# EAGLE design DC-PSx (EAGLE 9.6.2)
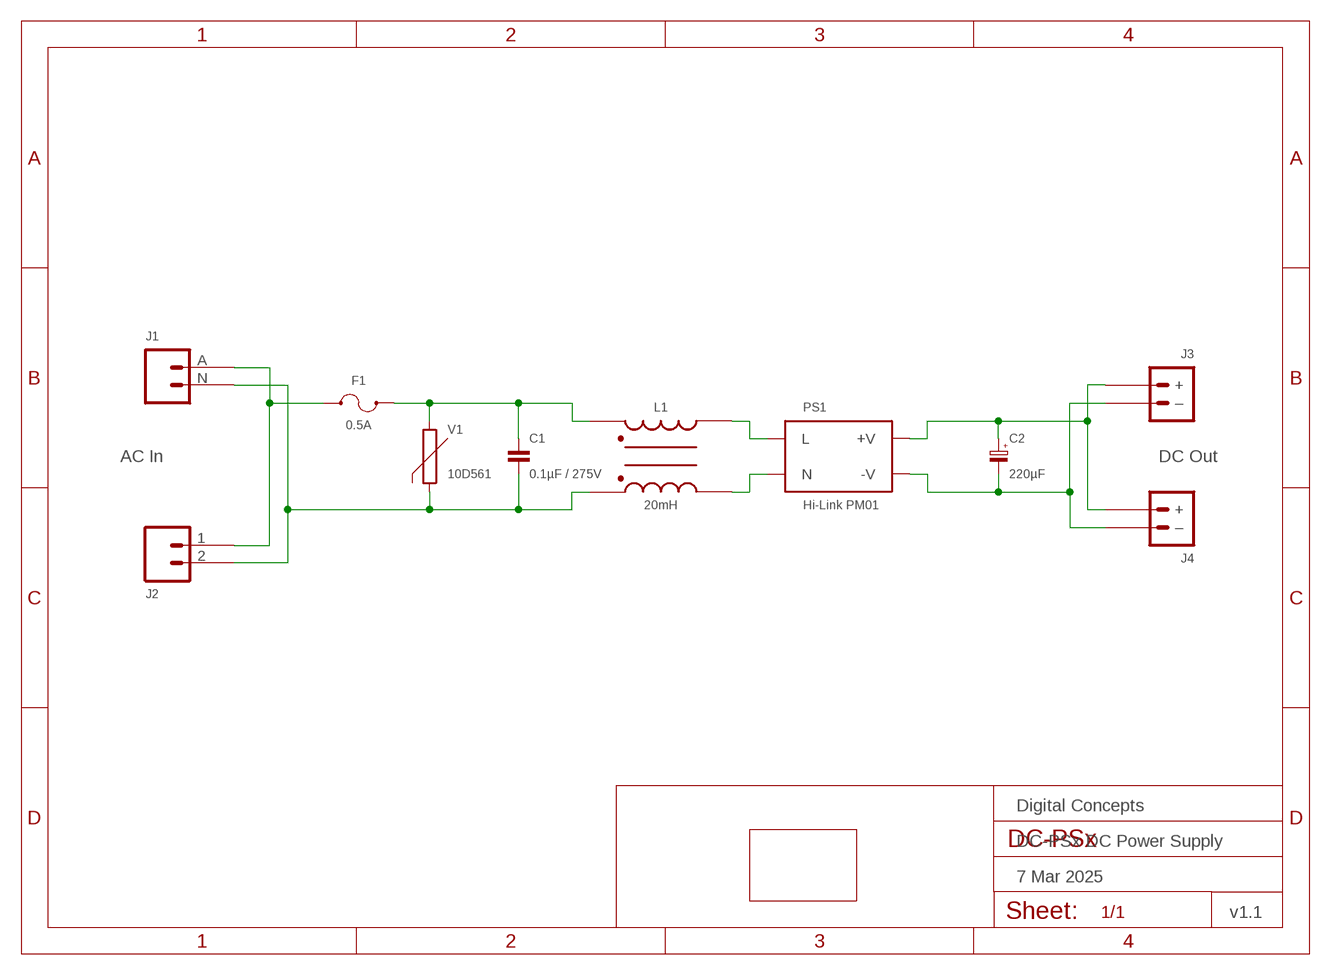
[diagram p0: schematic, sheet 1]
FRAME2 (FRAME_A5L-LOC): DATE: 7 Mar 2025; OWNER: Digital Concepts; TITLE: DC-PSx DC Power Supply; VERSION: v1.1

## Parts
C1  0.1µF / 275V  CAPACITOR-TENTA-SUPPRESSION  [CAPACITOR-TENTA-SUPPRESSION]
C2  220µF  CAPACITOR-ELECTROLYTICE5-10.5  [E5-10,5]
F1  0.5A  FUSE-HOLDER-1808  [FUSE-HOLDER-1808]
J1  AC In  AC_POWER_SOCKET_DB-03  [DB-03_AC_POWER_SOCKET]
J2  TERMINAL_SCREW_2P_VERTICAL  [TERMINAL-SCREW-2P]
J3  DC Out  JST-PH2.0-2-VERTICAL-POWER  [JST-PH2.0-2-VERTICAL-POWER]
J4  TERMINAL_SCREW_2P_POWER  [TERMINAL-SCREW-2P]
L1  20mH  INDUCTOR-COMMON-MODE-UU9.8  [INDUCTOR-UU9.8]
PCB1  PCB-OUTLINE-64X36  [PCB-POWER-SUPPLY-3]
PS1  Hi-Link PM01  POWER_SUPPLY-HI-LINK  [HI-LINK_PM0X]
V1  10D561  VARISTOR-10D561  [VARISTOR-10D561]

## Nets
N$1: F1.P$1 J1.A J2.1
N$2: C1.P$1 F1.P$2 L1.P$1 V1.2
N$3: L1.P$2 PS1.AC-L(L)
N$4: C1.P$2 J1.N J2.2 L1.P$4 V1.1
N$5: L1.P$3 PS1.AC-N(N)
N$6: C2.+ J3.+ J4.2(+) PS1.+VO(+V)
N$7: C2.- J3.-(–) J4.1(–) PS1.-VO(-V)

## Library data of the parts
C1 = digitalconcepts:CAPACITOR-TENTA-SUPPRESSION: MEX/TENTA Interference Suppression Capacitor
C2 = digitalconcepts:CAPACITOR-ELECTROLYTIC: Electrolytic Capacitor; SPICEPREFIX: C
F1 = digitalconcepts:FUSE-HOLDER-1808: 1808 Fuse Holder
J1 = digitalconcepts:AC_POWER_SOCKET_DB-03: DB-03 AC Power Socket
J2 = digitalconcepts:TERMINAL_SCREW_2P_VERTICAL: PCB Mount Screw-Type Terminal 2P
J3 = digitalconcepts:JST-PH2.0-2-VERTICAL-POWER: JST PH2.0 2P PTH Connector (Power)
J4 = digitalconcepts:TERMINAL_SCREW_2P_POWER: PCB Mount Screw-Type Terminal 2P
L1 = digitalconcepts:INDUCTOR-COMMON-MODE-UU9.8: UU9.8 Common Mode Inductor
PCB1 = digitalconcepts:PCB-OUTLINE-64X36: Power Supply PCB Outline (64 x 36)
PS1 = digitalconcepts:POWER_SUPPLY-HI-LINK: Hi-Link Power Supply Module
V1 = digitalconcepts:VARISTOR-10D561: VARISTOR

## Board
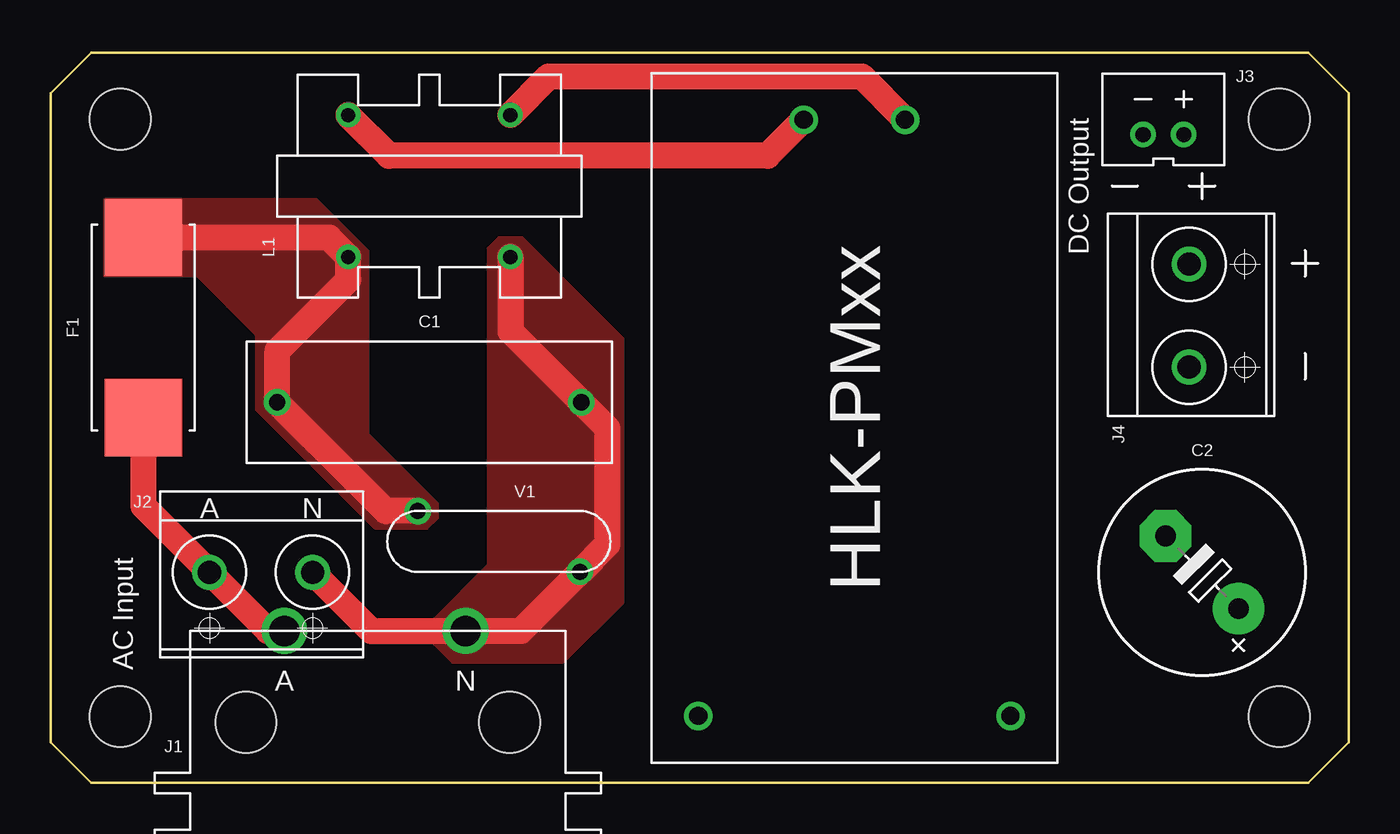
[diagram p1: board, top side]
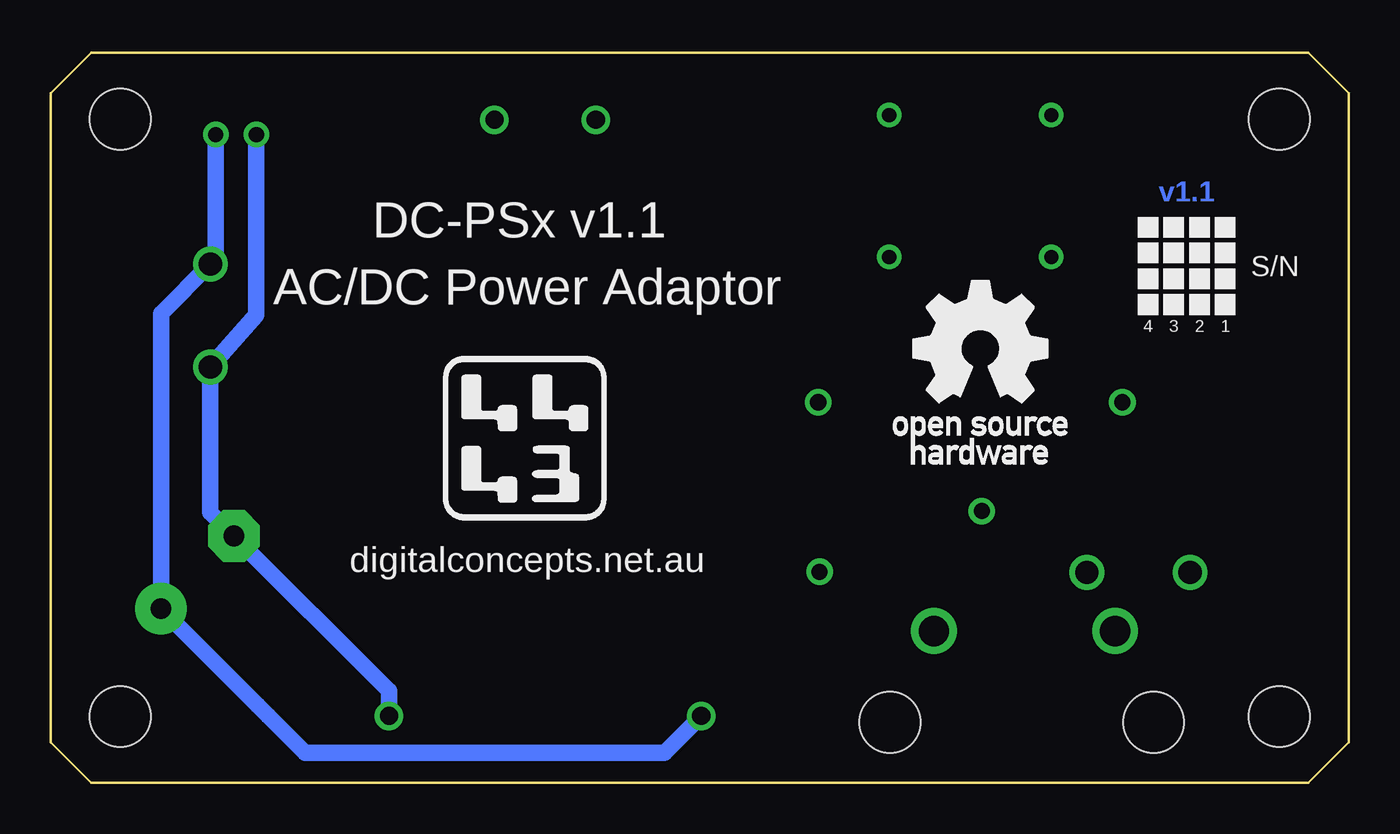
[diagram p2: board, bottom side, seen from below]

Size 64 x 36 mm. Coordinates in mm from the lower left corner, seen from the top.
Copper layers (1*16): Top 0.035mm / dielectric 1.5mm / Bottom 0.035mm
Design rules "default *": minimum track width 6mil, minimum drill 0.35mm, track to track 6mil, track to pad 6mil, pad to pad 6mil, via to via 6mil, smd to smd 6mil, copper to edge 6mil, drill to drill 6mil, minimum pad ring 10mil, minimum via ring 8mil, stop-mask expansion 4mil, vias tented up to drill 0mil, thermal gap 10mil

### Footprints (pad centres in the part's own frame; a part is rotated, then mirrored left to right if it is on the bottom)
CAPACITOR-TENTA-SUPPRESSION = drill 0.8: P$1 -7.5,0; P$2 7.5,0
E5-10,5 = drill 1.016 pad 2.54: + -2.54,0 | drill 1.016 pad 2.54 octagon: - 2.54,0
FUSE-HOLDER-1808 = smd 3.81 x 3.81: P$1 -4.445,0; P$2 4.445,0
DB-03_AC_POWER_SOCKET = drill 1.5: A 4.6,-6; N -4.33,-6 | hole 3: -6.5,-1.5; 6.5,-1.5
TERMINAL-SCREW-2P = drill 1.143: 1 -2.58,0; 2 2.5,0
JST-PH2.0-2-VERTICAL-POWER = drill 0.75: + -1,0; - 1,0
INDUCTOR-UU9.8 = drill 0.7: P$1 -3.5,4; P$2 3.5,4; P$3 3.5,-4; P$4 -3.5,-4
PCB-POWER-SUPPLY-3 = hole 3: -28.575,14.732; -28.575,-14.732; 28.575,-14.732; 28.575,14.732
HI-LINK_PM0X = drill 0.9: +VO 14.7,-7.7; -VO 14.7,7.7; AC-L -14.7,-2.5; AC-N -14.7,2.5
VARISTOR-10D561 = drill 0.8: 1 -4,1.5; 2 4,-1.5

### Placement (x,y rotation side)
C1  18.66,18.76 0 top
C2  56.77,10.38 135 top
F1  4.57,22.45 90 top
J1  16.12,1.49 180 top
J2  10.41,10.38 0 top
J3  54.86,31.97 180 top
J4  56.13,23.08 90 top
L1  18.66,29.43 90 top
PCB1  32,18 0 top
PS1  39.62,18 270 top
V1  22.09,11.9 180 top

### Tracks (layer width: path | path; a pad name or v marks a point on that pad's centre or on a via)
N$1
  Top 1.27: 5.29,18 F1.P$1 4.57,13.64 J2.1 10.72,7.49 J1.A
N$2
  Top 1.27: V1.2 16.52,13.4 C1.P$1 11.16,21.3 14.66,24.8 L1.P$1 13.7,26.89 F1.P$2
  pour Top (no thermals): 2.66,28.8 13.08,28.8 15.62,26.26 15.62,17.24 19.05,13.81 19.05,13.05 18.54,12.54 16,12.54 10.16,18.38 10.16,22.06 7.23,24.98 2.66,24.98
N$3
  Top 1.27: L1.P$2 16.67,30.92 35.34,30.92 PS1.AC-L
N$4
  Top 1.27: L1.P$4 22.66,22.26 C1.P$2 27.43,17.49 27.43,11.75 V1.1 23.18,7.49 J1.N 15.8,7.49 J2.2
  pour Top (no thermals): 22.09,26.89 23.24,26.89 28.19,21.94 28.19,8.86 25.27,5.94 19.81,5.94 18.92,6.82 18.92,8.09 21.59,10.76 21.59,26.38
N$5
  Top 1.27: L1.P$3 24.57,34.84 39.98,34.84 PS1.AC-N
N$6
  Bottom 0.813: J3.+ 55.86,25.85 J4.2 58.56,23.15 C2.+ 53.8,3.82 53.28,3.3 51.47,1.49 33.73,1.49 PS1.+VO
N$7
  Bottom 0.813: J3.- 53.86,23.08 J4.1 56.13,13.34 C2.- 47.32,4.53 PS1.-VO

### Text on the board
Bottom: v1.1
tPlace: A | N | A | N
bPlace: DC-PSx v1.1 | S/N | AC/DC Power Adaptor | 1 | 2 | 3 | 4 | digitalconcepts.net.au
tNames: DC Output | AC Input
